ORGANIZATION_BLOCK OB 1
BEGIN

	// Test C# immediate
	L		C#123
	__ASSERT==	__ACCU 1,	291


	// Test down counter (ZR)
	CLR
	FR		Z 10
	SET
	R		Z 10
	FR		Z 10
	U		Z 10
	__ASSERT==	__STW VKE,	0
	L		C#123
	SET
	S		Z 10
	U		Z 10
	__ASSERT==	__STW VKE,	1
	CLR
	ZR		Z 10
	U		Z 10
	__ASSERT==	__STW VKE,	1
	L		Z 10
	__ASSERT==	__ACCU 1,	123
	SET
	ZR		Z 10
	U		Z 10
	__ASSERT==	__STW VKE,	1
	L		Z 10
	__ASSERT==	__ACCU 1,	122
	CLR
	ZR		Z 10
	U		Z 10
	__ASSERT==	__STW VKE,	1
	L		Z 10
	__ASSERT==	__ACCU 1,	122
	LC		Z 10
	__ASSERT==	__ACCU 1,	C#122
	L		C#1
	CLR
	S		Z 10
	SET
	S		Z 10
	U		Z 10
	__ASSERT==	__STW VKE,	1
	L		Z 10
	__ASSERT==	__ACCU 1,	1
	CLR
	ZR		Z 10
	U		Z 10
	__ASSERT==	__STW VKE,	1
	SET
	ZR		Z 10
	U		Z 10
	__ASSERT==	__STW VKE,	0
	L		Z 10
	__ASSERT==	__ACCU 1,	0
	CLR
	ZR		Z 10
	U		Z 10
	__ASSERT==	__STW VKE,	0
	SET
	ZR		Z 10
	U		Z 10
	__ASSERT==	__STW VKE,	0
	L		Z 10
	__ASSERT==	__ACCU 1,	0


	// Test up counter (ZV)
	CLR
	FR		Z 10
	SET
	R		Z 10
	FR		Z 10
	U		Z 10
	__ASSERT==	__STW VKE,	0
	L		C#123
	SET
	S		Z 10
	U		Z 10
	__ASSERT==	__STW VKE,	1
	CLR
	ZV		Z 10
	U		Z 10
	__ASSERT==	__STW VKE,	1
	L		Z 10
	__ASSERT==	__ACCU 1,	123
	SET
	ZV		Z 10
	U		Z 10
	__ASSERT==	__STW VKE,	1
	L		Z 10
	__ASSERT==	__ACCU 1,	124
	CLR
	ZV		Z 10
	U		Z 10
	__ASSERT==	__STW VKE,	1
	L		Z 10
	__ASSERT==	__ACCU 1,	124
	LC		Z 10
	__ASSERT==	__ACCU 1,	C#124
	L		C#998
	CLR
	S		Z 10
	SET
	S		Z 10
	U		Z 10
	__ASSERT==	__STW VKE,	1
	L		Z 10
	__ASSERT==	__ACCU 1,	998
	CLR
	ZV		Z 10
	U		Z 10
	__ASSERT==	__STW VKE,	1
	SET
	ZV		Z 10
	U		Z 10
	__ASSERT==	__STW VKE,	1
	L		Z 10
	__ASSERT==	__ACCU 1,	999
	CLR
	ZV		Z 10
	U		Z 10
	__ASSERT==	__STW VKE,	1
	SET
	ZV		Z 10
	U		Z 10
	__ASSERT==	__STW VKE,	1
	L		Z 10
	__ASSERT==	__ACCU 1,	999


	// Test FR
	CLR
	FR		Z 10
	SET
	R		Z 10
	FR		Z 10
	U		Z 10
	__ASSERT==	__STW VKE,	0
	SET
	ZV		Z 10
	L		Z 10
	__ASSERT==	__ACCU 1,	1
	CLR
	FR		Z 10
	SET
	FR		Z 10
	ZV		Z 10
	L		Z 10
	__ASSERT==	__ACCU 1,	2
	ZR		Z 10
	L		Z 10
	__ASSERT==	__ACCU 1,	1
	CLR
	FR		Z 10
	SET
	FR		Z 10
	ZR		Z 10
	L		Z 10
	__ASSERT==	__ACCU 1,	0
	SET
	L		C#321
	S		Z 10
	L		Z 10
	__ASSERT==	__ACCU 1,	321
	CLR
	FR		Z 10
	SET
	FR		Z 10
	L		C#123
	S		Z 10
	L		Z 10
	__ASSERT==	__ACCU 1,	123
	SET
	FR		Z 10
	L		C#888
	S		Z 10
	L		Z 10
	__ASSERT==	__ACCU 1,	123


	// Test counter parameter
	AUF		DB 1
	L		DBW 0
	__ASSERT==	__ACCU 1,	24
	CALL FB 1, DB 1 (
		COUNTER_VAR	:= Z 42
	)


	CALL SFC 46 // STOP CPU
END_ORGANIZATION_BLOCK


FUNCTION_BLOCK FB 1
	VAR_INPUT
		COUNTER_VAR	: COUNTER
	END_VAR
BEGIN
	L		DIW 0
	__ASSERT==	__ACCU 1,	42
	L		#COUNTER_VAR
	__ASSERT==	__ACCU 1,	0
	U		#COUNTER_VAR
	__ASSERT==	__STW VKE,	0
	SET
	ZV		Z 42
	CLR
	ZV		Z 42
	U		#COUNTER_VAR
	__ASSERT==	__STW VKE,	1
	L		#COUNTER_VAR
	__ASSERT==	__ACCU 1,	1

	ZV		#COUNTER_VAR
	ZR		#COUNTER_VAR
	FR		#COUNTER_VAR
END_FUNCTION_BLOCK


DATA_BLOCK DB 1
	FB 1
BEGIN
	COUNTER_VAR	:= Z 24
END_DATA_BLOCK
